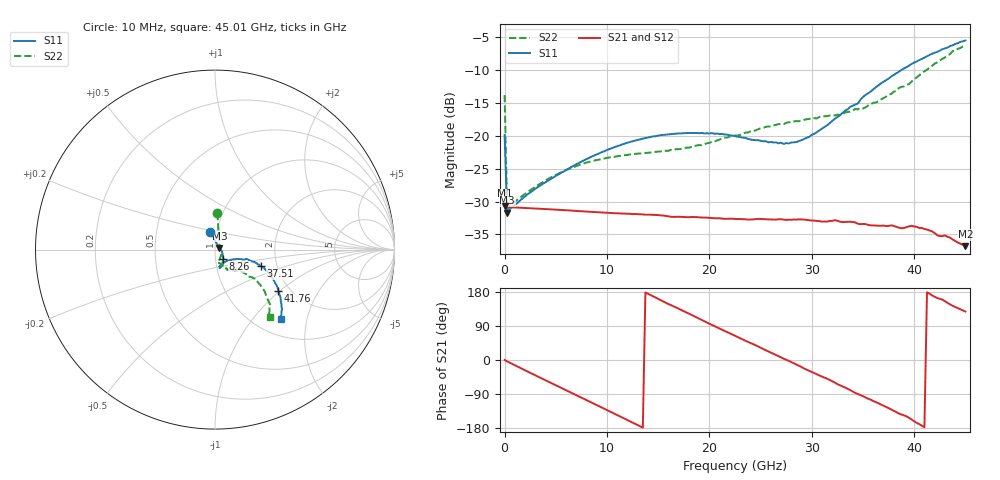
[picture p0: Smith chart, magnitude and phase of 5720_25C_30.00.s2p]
! Device:  ADRF5720
! Description: 0.5dB LSB GaAs MMIC 6-bit Digital Attenuator
! Frequency:  0.000009 -  40 GHz
! Ports:
!	RF1	= Port 1
!	RF2	= Port 2
! Vdd:  3.3 Volt
! Vss:  -3.3 Volt
! Control:  0/3.3 Volt
! State:  30.00 dB attenuation
! Data:  The device was measured using G-S-G Probes on a matrix board.
!  Data was collected using an calibrated 4 port network analyzer.
!  The reference plane for this measurement is at the launchers.
! Note:  Analog Devices supplies this data as a sample of measured data
!  for this product.  Your particular data for this product may vary.
!  Data was taken at 25 degrees C.
!  Analog Devices reserves the right to change this data at anytime.
# GHZ S DB R 45.0
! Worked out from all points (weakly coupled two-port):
!   181 points, 10 MHz to 45.01 GHz, reference 45 ohm
!   highest |S21| = -30.64 dB at 10 MHz (marker M1); lowest = -36.8 dB at 45.01 GHz (marker M2)
!   lowest |S11| = -31.7 dB at 260 MHz (marker M3), VSWR 1.05, Z = 47.2 + j0.882 ohm
!   |S11| at or under -10 dB: start of sweep to 38.75 GHz
!   |S22| runs from -31.3 to -6.2 dB; largest |S21 - S12| = 0.00012
!   S11 on the Smith chart (normalised r, x): 10 MHz: 0.93, +0.18; 8.26 GHz: 1.09, -0.11; 37.51 GHz: 1.65, -0.33; 41.76 GHz: 1.75, -0.97; 45.01 GHz: 1.30, -1.40
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0.01  -19.87 106.9  -30.64 0.1  -30.63 0.1  -13.80 86.3
0.26  -31.71 21.1  -30.83 -3.7  -30.84 -3.7  -31.32 17.3
0.51  -31.19 11.8  -30.85 -7.1  -30.86 -7.1  -30.64 7.1
3.26  -27.78 -17.5  -31.08 -43.7  -31.07 -43.7  -27.48 -34.1
7.76  -23.73 -46.2  -31.49 -102.7  -31.49 -102.6  -24.19 -67.1
8.26  -23.35 -48.5  -31.54 -109.2  -31.54 -109.1  -23.98 -68.9
12.01  -21.04 -62.0  -31.85 -158.4  -31.85 -158.4  -22.91 -77.0
15.26  -19.90 -69.9  -32.10 157.8  -32.10 157.8  -22.37 -76.1
20.26  -19.58 -75.9  -32.50 92.4  -32.50 92.4  -20.94 -66.3
22.76  -20.14 -75.0  -32.66 60.6  -32.66 60.7  -19.95 -62.3
27.26  -21.24 -56.3  -32.74 3.4  -32.73 3.5  -18.23 -58.6
28.51  -20.95 -46.9  -32.74 -12.1  -32.73 -12.1  -17.77 -58.9
30.26  -19.68 -33.5  -32.89 -34.5  -32.90 -34.5  -17.32 -56.7
34.51  -15.07 -17.3  -33.37 -89.9  -33.34 -89.9  -15.98 -47.7
35.01  -14.10 -17.1  -33.40 -95.5  -33.40 -95.4  -15.85 -46.3
37.51  -11.29 -19.7  -33.70 -126.9  -33.71 -126.8  -13.77 -39.0
37.76  -10.99 -20.3  -33.61 -130.4  -33.60 -130.3  -13.64 -38.5
39.01  -9.75 -23.4  -34.02 -146.1  -34.04 -145.9  -12.48 -39.0
39.76  -9.07 -26.1  -33.69 -157.1  -33.65 -157.2  -11.75 -36.6
41.76  -7.52 -32.9  -34.53 170.5  -34.50 170.6  -9.37 -39.1
43.76  -6.24 -40.6  -35.76 143.1  -35.73 143.2  -7.11 -45.3
45.01  -5.50 -46.6  -36.78 127.9  -36.75 127.9  -6.23 -50.7
